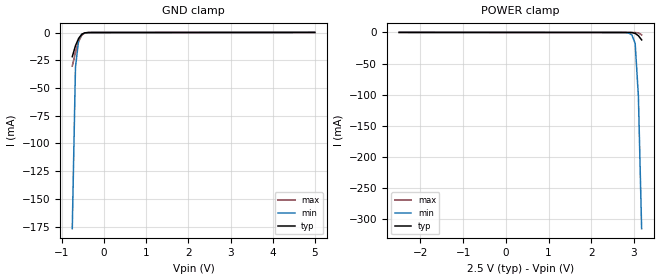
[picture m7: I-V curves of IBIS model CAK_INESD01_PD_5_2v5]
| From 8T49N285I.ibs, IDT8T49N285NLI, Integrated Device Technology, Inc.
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[Model] CAK_INESD01_PD_5_2v5
Model_type   Input
Polarity   Non-Inverting
Vinl = 0.7V
Vinh = 1.7V
|   typ   min   max
C_comp   2pF   1.5pF   2.5pF
|   typ   min   max
[Voltage range]   2.5V   2.375V   2.625V
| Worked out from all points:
|   GND clamp passes 1 mA (typ) near -0.50 V on its own axis
[GND_clamp]
|Voltage   I (typ)   I (min)   I (max)
|Note, modeling breaks down at 250mA and above.  This is well beyond the functional   |
|operating range of the device.  Should this scenario occur, catastrophic failure and   |
|possible damage to the device and/or board is of higher concern than the I-V curve   |
|behavior.  The IBIS checker will flag currents in excess of 10A with warnings.  Lines   |
|with currents in excess of 0.35 A have been commented out.  The points still remain|
|available to the user if the user desires to use them.   |
|-2.50000e+00   -6.31277e+00   -5.12658e+00   -7.65734e+00
|-2.42424e+00   -6.02353e+00   -4.90997e+00   -7.28820e+00
|-2.34848e+00   -5.73432e+00   -4.69344e+00   -6.91907e+00
|-2.27273e+00   -5.44517e+00   -4.47699e+00   -6.54996e+00
|-2.19697e+00   -5.15608e+00   -4.26064e+00   -6.18087e+00
|-2.12121e+00   -4.86706e+00   -4.04438e+00   -5.81182e+00
|-2.04545e+00   -4.57811e+00   -3.82823e+00   -5.44281e+00
|-1.96970e+00   -4.28924e+00   -3.61218e+00   -5.07385e+00
|-1.89394e+00   -4.00047e+00   -3.39625e+00   -4.70495e+00
|-1.81818e+00   -3.71181e+00   -3.18045e+00   -4.33613e+00
|-1.74242e+00   -3.42327e+00   -2.96477e+00   -3.96740e+00
|-1.66667e+00   -3.13486e+00   -2.74923e+00   -3.59876e+00
|-1.59091e+00   -2.84661e+00   -2.53383e+00   -3.23023e+00
|-1.51515e+00   -2.55852e+00   -2.31859e+00   -2.86183e+00
|-1.43939e+00   -2.27062e+00   -2.10350e+00   -2.49356e+00
|-1.36364e+00   -1.98293e+00   -1.88857e+00   -2.12547e+00
|-1.28788e+00   -1.69546e+00   -1.67382e+00   -1.75758e+00
|-1.21212e+00   -1.40825e+00   -1.45924e+00   -1.38992e+00
|-1.13636e+00   -1.12130e+00   -1.24485e+00   -1.02253e+00
|-1.06061e+00   -8.34641e-01   -1.03066e+00   -6.55447e-01
|-9.84848e-01   -5.48303e-01   -8.16729e-01   -2.88713e-01
|-9.09091e-01   -2.62314e-01   -6.03115e-01   -6.18263e-02
|-8.33333e-01   -5.02723e-02   -3.89971e-01   -4.19557e-02
-757.6mV  -21.77mA   -176.8mA   -30.29mA
-681.8mV  -11.94mA   -31.43mA   -17.97mA
-606.1mV  -5.237mA   -6.649mA   -8.121mA
-530.3mV  -1.497mA   -1.616mA   -2.258mA
-454.5mV  -253.9uA   -336.2uA   -326.7uA
-378.8mV  -33.3uA    -60.54uA   -32.84uA
5V        99.6uA     87.28uA    115.1uA
[Power_clamp]
|Voltage   I (typ)   I (min)   I (max)
|Note, modeling breaks down at 250mA and above.  This is well beyond the functional   |
|operating range of the device.  Should this scenario occur, catastrophic failure and   |
|possible damage to the device and/or board is of higher concern than the I-V curve   |
|behavior.  The IBIS checker will flag currents in excess of 10A with warnings.  Lines   |
|with currents in excess of 0.35 A have been commented out.  The points still remain|
|available to the user if the user desires to use them.   |
-2.5V     99.6uA     85.1uA     117.9uA
2.727V    -4.634uA   -33.61uA   -2.354uA
2.879V    -33.3uA    -955.9uA   -5.936uA
2.955V    -253.9uA   -4.064mA   -10.75uA
3.03V     -1.497mA   -17.62mA   -73.27uA
3.106V    -5.237mA   -102.4mA   -686.5uA
3.182V    -11.94mA   -315.5mA   -3.8mA
